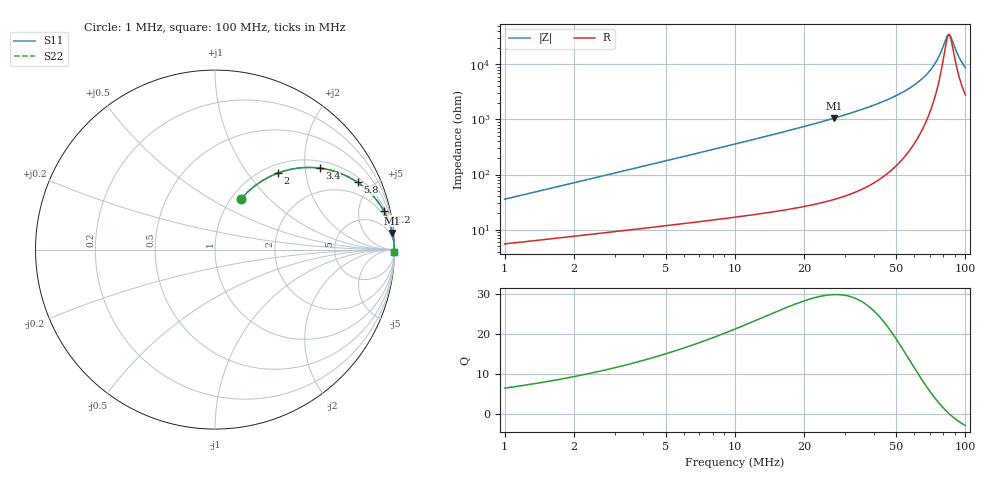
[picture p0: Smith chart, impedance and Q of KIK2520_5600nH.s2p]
!version-2
!date-01.2022
!Series
# MHz S RI R 50
!Freq ReS11 ImS11 ReS21 ImS21 ReS12 ImS12 ReS22 ImS22
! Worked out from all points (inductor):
!   496 points, 1 MHz to 100 MHz, reference 50 ohm
!   read as one part in series: L = 5.6 uH near 1.4 MHz
!   highest Q = 29.9 at 27 MHz (marker M1), where L = 6.23 uH
!   self-resonance near 84.8 MHz
!   S11 on the Smith chart (normalised r, x): 1 MHz: 1.11, +0.70; 2 MHz: 1.15, +1.41; 3.4 MHz: 1.19, +2.40; 5.8 MHz: 1.25, +4.10; 12.2 MHz: 1.38, +8.77; 100 MHz: open
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1  0.147 0.2845  0.853 -0.2845  0.853 -0.2845  0.147 0.2845
2  0.3492 0.4259  0.6508 -0.4259  0.6508 -0.4259  0.3492 0.4259
2.6  0.4618 0.4539  0.5382 -0.4539  0.5382 -0.4539  0.4618 0.4539
3.4  0.5843 0.4538  0.4157 -0.4538  0.4157 -0.4538  0.5843 0.4538
4.6  0.7127 0.4191  0.2873 -0.4191  0.2873 -0.4191  0.7127 0.4191
5.8  0.7942 0.3746  0.2058 -0.3746  0.2058 -0.3746  0.7942 0.3746
8.4  0.8874 0.2915  0.1126 -0.2915  0.1126 -0.2915  0.8874 0.2915
12.2  0.9424 0.2125  0.0576 -0.2125  0.0576 -0.2125  0.9424 0.2125
17.6  0.9715 0.1491  0.0285 -0.1491  0.0285 -0.1491  0.9715 0.1491
27  0.9881 0.0931  0.0119 -0.0931  0.0119 -0.0931  0.9881 0.0931
34  0.9927 0.0694  0.00729 -0.0694  0.00729 -0.0694  0.9927 0.0694
50.6  0.9967 0.036  0.00326 -0.036  0.00326 -0.036  0.9967 0.036
59.8  0.9974 0.0238  0.00261 -0.0238  0.00261 -0.0238  0.9974 0.0238
67  0.9975 0.0159  0.00246 -0.0159  0.00246 -0.0159  0.9975 0.0159
71.6  0.9975 0.0114  0.00247 -0.0114  0.00247 -0.0114  0.9975 0.0114
75.4  0.9975 0.00791  0.00254 -0.00791  0.00254 -0.00791  0.9975 0.00791
83.6  0.9972 0.00105  0.00281 -0.00105  0.00281 -0.00105  0.9972 0.00105
84.8  0.9971 0.000105  0.00286 -0.000105  0.00286 -0.000105  0.9971 0.000105
86  0.9971 -0.000825  0.00292 0.000825  0.00292 0.000825  0.9971 -0.000825
93.2  0.9967 -0.00614  0.00332 0.00614  0.00332 0.00614  0.9967 -0.00614
96.6  0.9965 -0.00852  0.00354 0.00852  0.00354 0.00852  0.9965 -0.00852
100  0.9962 -0.0108  0.00378 0.0108  0.00378 0.0108  0.9962 -0.0108
